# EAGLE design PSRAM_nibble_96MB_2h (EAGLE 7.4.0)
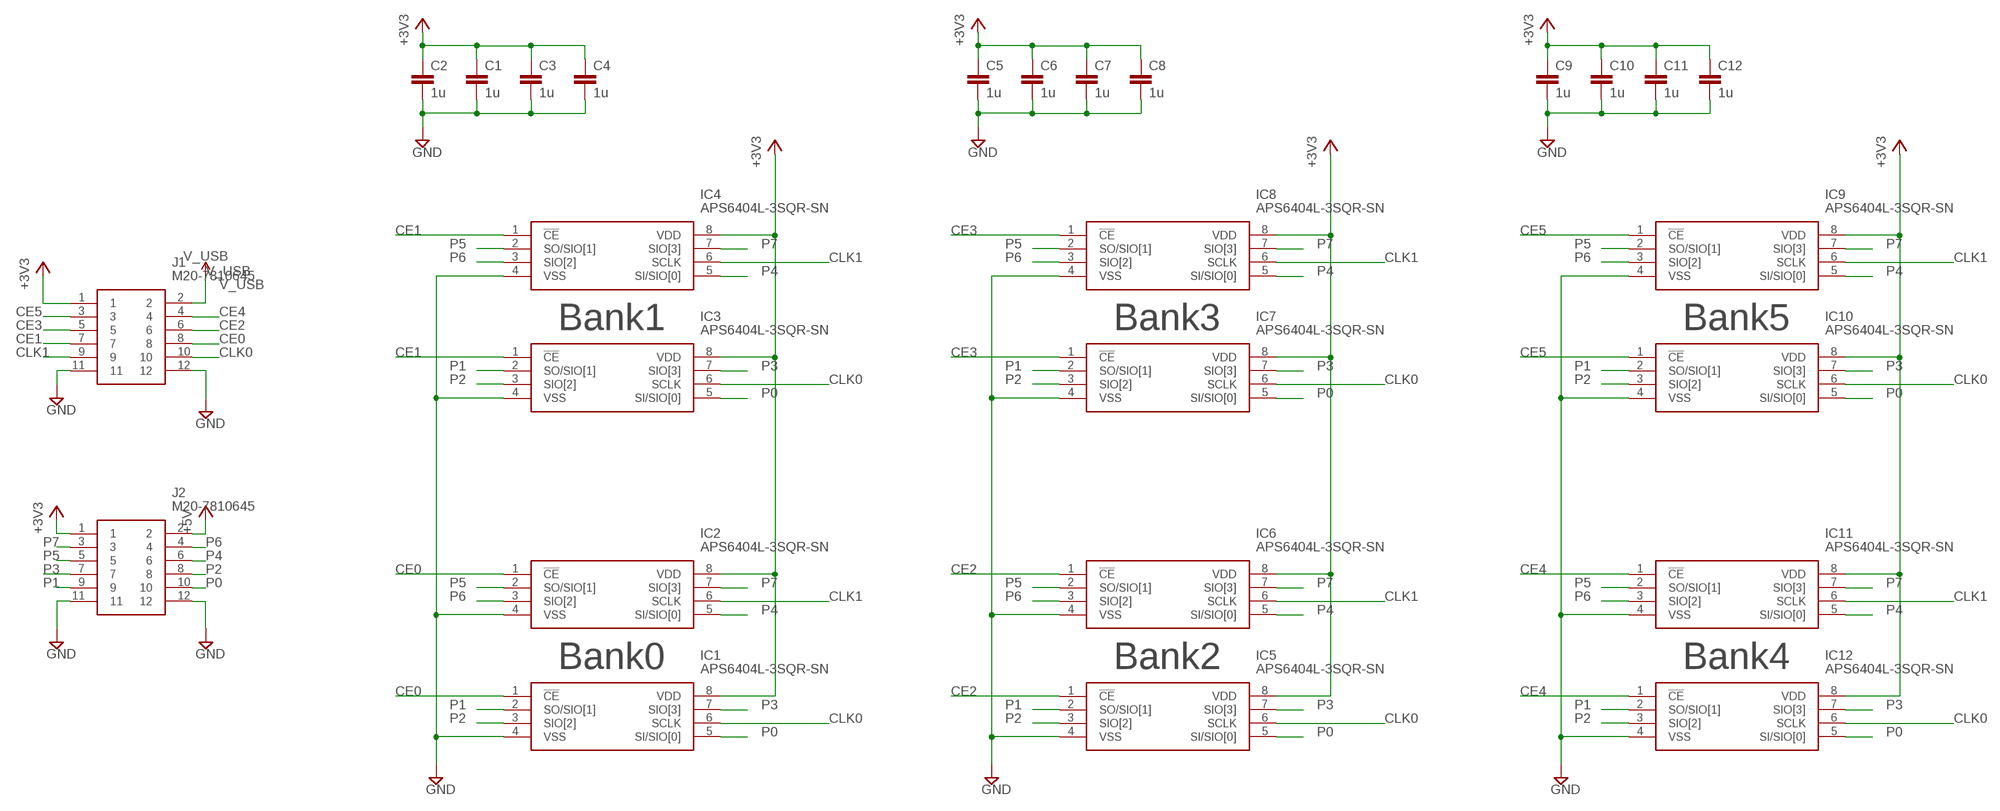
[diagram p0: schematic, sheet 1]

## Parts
C1  1u  1.0UF-25V-+80/-20(0805)  [0805@1]
C2  1u  1.0UF-25V-+80/-20(0805)  [0805@1]
C3  1u  1.0UF-25V-+80/-20(0805)  [0805@1]
C4  1u  1.0UF-25V-+80/-20(0805)  [0805@1]
C5  1u  1.0UF-25V-+80/-20(0805)  [0805@1]
C6  1u  1.0UF-25V-+80/-20(0805)  [0805@1]
C7  1u  1.0UF-25V-+80/-20(0805)  [0805@1]
C8  1u  1.0UF-25V-+80/-20(0805)  [0805@1]
C9  1u  1.0UF-25V-+80/-20(0805)  [0805@1]
C10  1u  1.0UF-25V-+80/-20(0805)  [0805@1]
C11  1u  1.0UF-25V-+80/-20(0805)  [0805@1]
C12  1u  1.0UF-25V-+80/-20(0805)  [0805@1]
IC1  APS6404L-3SQR-SN  [SOIC127P600X175-8N]
IC2  APS6404L-3SQR-SN  [SOIC127P600X175-8N]
IC3  APS6404L-3SQR-SN  [SOIC127P600X175-8N]
IC4  APS6404L-3SQR-SN  [SOIC127P600X175-8N]
IC5  APS6404L-3SQR-SN  [SOIC127P600X175-8N]
IC6  APS6404L-3SQR-SN  [SOIC127P600X175-8N]
IC7  APS6404L-3SQR-SN  [SOIC127P600X175-8N]
IC8  APS6404L-3SQR-SN  [SOIC127P600X175-8N]
IC9  APS6404L-3SQR-SN  [SOIC127P600X175-8N]
IC10  APS6404L-3SQR-SN  [SOIC127P600X175-8N]
IC11  APS6404L-3SQR-SN  [SOIC127P600X175-8N]
IC12  APS6404L-3SQR-SN  [SOIC127P600X175-8N]
J1  M20-7810645  [M207810645]
J2  M20-7810645  [M207810645]

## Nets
+3V3: C1.1 C2.1 C3.1 C4.1 C5.1 C6.1 C7.1 C8.1 C9.1 C10.1 C11.1 C12.1 IC1.8(VDD) IC2.8(VDD) IC3.8(VDD) IC4.8(VDD) IC5.8(VDD) IC6.8(VDD) IC7.8(VDD) IC8.8(VDD) IC9.8(VDD) IC10.8(VDD) IC11.8(VDD) IC12.8(VDD) J1.1 J2.1
+5V: J2.2
CE0: IC1.1(!CE) IC2.1(!CE) J1.8
CE1: IC3.1(!CE) IC4.1(!CE) J1.7
CE2: IC5.1(!CE) IC6.1(!CE) J1.6
CE3: IC7.1(!CE) IC8.1(!CE) J1.5
CE4: IC11.1(!CE) IC12.1(!CE) J1.4
CE5: IC9.1(!CE) IC10.1(!CE) J1.3
CLK0: IC1.6(SCLK) IC3.6(SCLK) IC5.6(SCLK) IC7.6(SCLK) IC10.6(SCLK) IC12.6(SCLK) J1.10
CLK1: IC2.6(SCLK) IC4.6(SCLK) IC6.6(SCLK) IC8.6(SCLK) IC9.6(SCLK) IC11.6(SCLK) J1.9
GND: C1.2 C2.2 C3.2 C4.2 C5.2 C6.2 C7.2 C8.2 C9.2 C10.2 C11.2 C12.2 IC1.4(VSS) IC2.4(VSS) IC3.4(VSS) IC4.4(VSS) IC5.4(VSS) IC6.4(VSS) IC7.4(VSS) IC8.4(VSS) IC9.4(VSS) IC10.4(VSS) IC11.4(VSS) IC12.4(VSS) J1.11 J1.12 J2.11 J2.12
P0: IC1.5(SI/SIO[0]) IC3.5(SI/SIO[0]) IC5.5(SI/SIO[0]) IC7.5(SI/SIO[0]) IC10.5(SI/SIO[0]) IC12.5(SI/SIO[0]) J2.10
P1: IC1.2(SO/SIO[1]) IC3.2(SO/SIO[1]) IC5.2(SO/SIO[1]) IC7.2(SO/SIO[1]) IC10.2(SO/SIO[1]) IC12.2(SO/SIO[1]) J2.9
P2: IC1.3(SIO[2]) IC3.3(SIO[2]) IC5.3(SIO[2]) IC7.3(SIO[2]) IC10.3(SIO[2]) IC12.3(SIO[2]) J2.8
P3: IC1.7(SIO[3]) IC3.7(SIO[3]) IC5.7(SIO[3]) IC7.7(SIO[3]) IC10.7(SIO[3]) IC12.7(SIO[3]) J2.7
P4: IC2.5(SI/SIO[0]) IC4.5(SI/SIO[0]) IC6.5(SI/SIO[0]) IC8.5(SI/SIO[0]) IC9.5(SI/SIO[0]) IC11.5(SI/SIO[0]) J2.6
P5: IC2.2(SO/SIO[1]) IC4.2(SO/SIO[1]) IC6.2(SO/SIO[1]) IC8.2(SO/SIO[1]) IC9.2(SO/SIO[1]) IC11.2(SO/SIO[1]) J2.5
P6: IC2.3(SIO[2]) IC4.3(SIO[2]) IC6.3(SIO[2]) IC8.3(SIO[2]) IC9.3(SIO[2]) IC11.3(SIO[2]) J2.4
P7: IC2.7(SIO[3]) IC4.7(SIO[3]) IC6.7(SIO[3]) IC8.7(SIO[3]) IC9.7(SIO[3]) IC11.7(SIO[3]) J2.3
V_USB: J1.2

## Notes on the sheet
- Bank1 | Bank3 | Bank5
- Bank0 | Bank2 | Bank4

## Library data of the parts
C1-C12 = SparkFun-Capacitors:1.0UF-25V-+80/-20(0805); PROD_ID: CAP-11625; VALUE: 1.0uF
IC1-IC12 = SamacSys_Parts:APS6404L-3SQR-SN: DRAM IoT RAM 64Mb QSPI (x1,x4) SDR 133/84MHz, RBX, 3V, Ind. Temp., SOP8 Source: Datasheet; DESCRIPTION: DRAM IoT RAM 64Mb QSPI (x1,x4) SDR 133/84MHz, RBX, 3V, Ind. Temp., SOP8; HEIGHT: 1.75mm; MANUFACTURER_NAME: AP Memory; MANUFACTURER_PART_NUMBER: APS6404L-3SQR-SN; MOUSER_PART_NUMBER: 878-APS6404L-3SQR-SN; MOUSER_PRICE-STOCK: https://www.mouser.co.uk/ProductDetail/AP-Memory/APS6404L-3SQR-SN?qs=IS%252B4QmGtzzqsn3S5xo%2FEEg%3D%3D
J1 J2 = SamacSys_Parts:M20-7810645: Headers & Wire Housings 6+6 DIL 2.54MM L/P SMT SKT Source: Datasheet; DESCRIPTION: Headers & Wire Housings 6+6 DIL 2.54MM L/P SMT SKT; HEIGHT: 3.7mm; MANUFACTURER_NAME: Harwin; MANUFACTURER_PART_NUMBER: M20-7810645; MOUSER_PART_NUMBER: 855-M20-7810645; MOUSER_PRICE-STOCK: https://www.mouser.co.uk/ProductDetail/Harwin/M20-7810645?qs=k41KVqW3ympKz0jQ%252Bxdz7A%3D%3D

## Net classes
1 power: width 0.254 mm
2 gnd: width 0.305 mm, drill 0.406 mm, clearance 0.203 mm

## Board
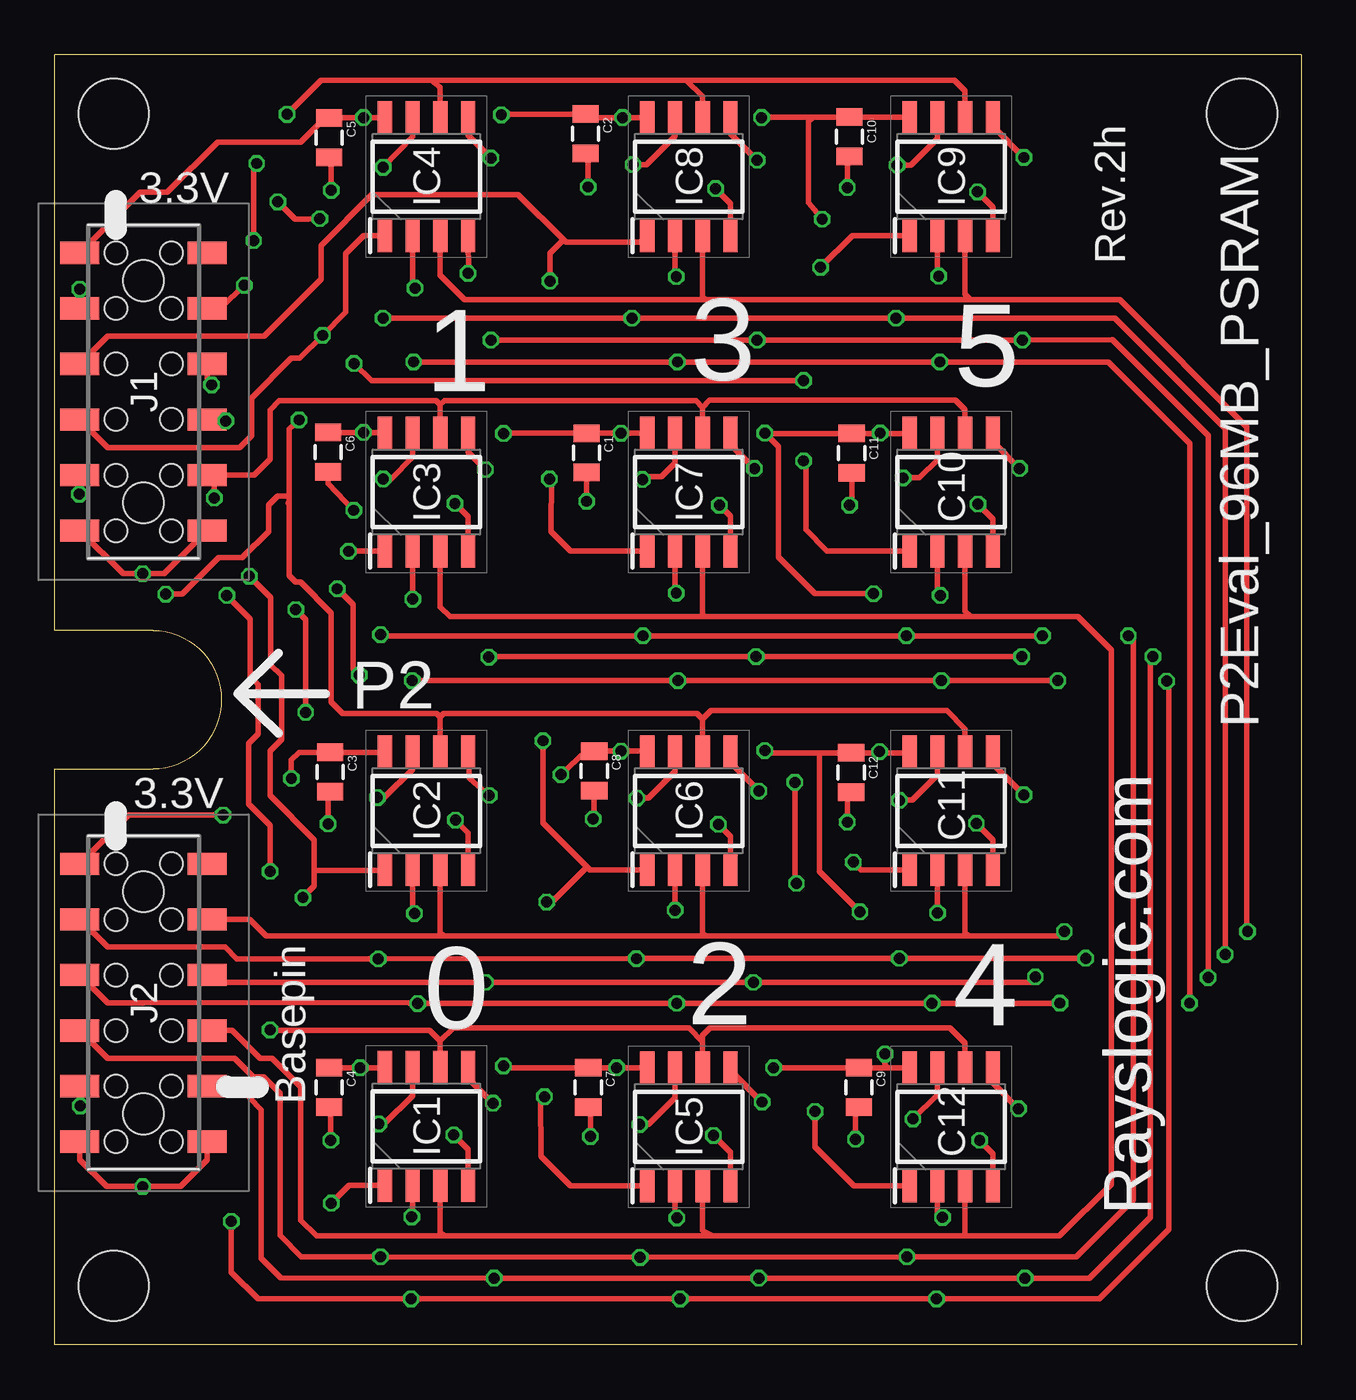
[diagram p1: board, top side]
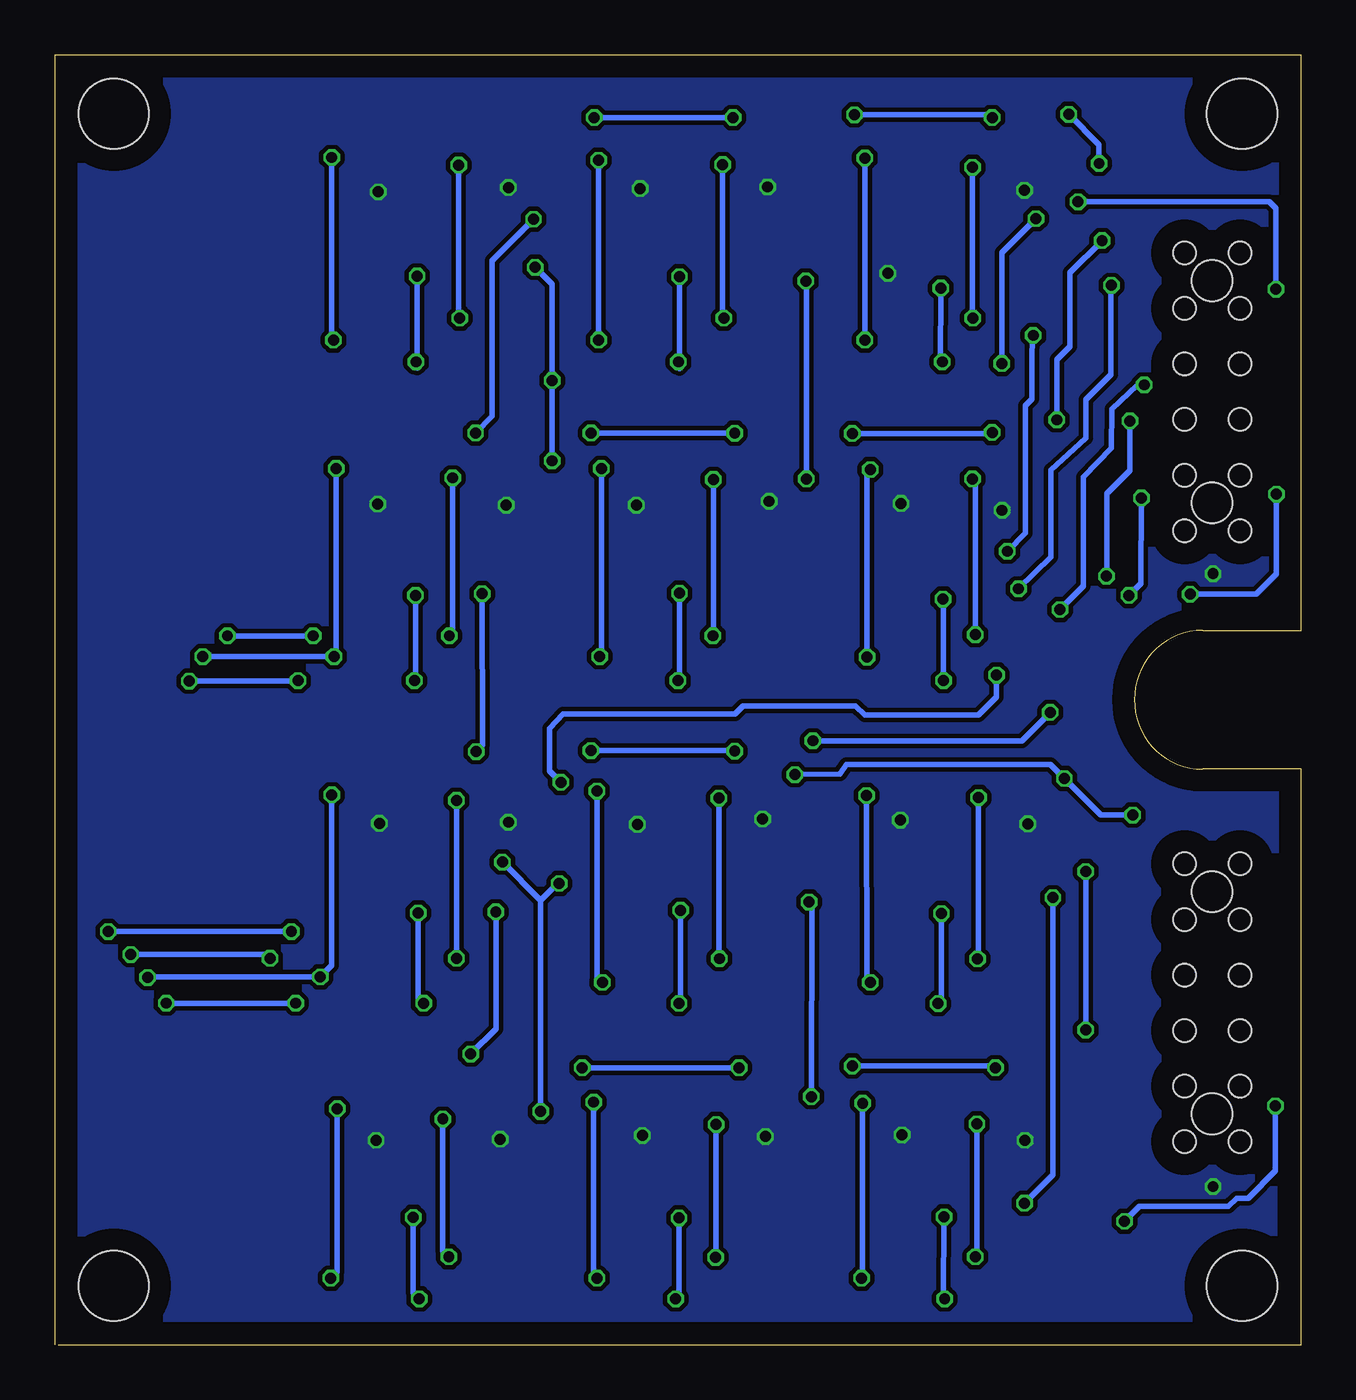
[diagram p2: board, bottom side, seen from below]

Size 57 x 59 mm. Coordinates in mm from the lower left corner, seen from the top.
Outline: 57,0 57,59 0,59 0,32.67 4.5,32.67 arc-90 7.62,29.5 arc-90 4.5,26.32 0,26.32 0,0 56.83,0
Copper layers (1*16): Top 0.035mm / dielectric 1.5mm / Bottom 0.035mm
Design rules "default *": minimum track width 10mil, minimum drill 8mil, track to track 8mil, track to pad 8mil, pad to pad 8mil, via to via 8mil, smd to smd 8mil, copper to edge 40mil, drill to drill 8mil, minimum pad ring 10mil, minimum via ring 4mil, stop-mask expansion 4mil, vias tented up to drill 0mil, thermal gap 10mil
Holes 3.2 mm at 2.7,56.3 54.3,56.3 2.7,2.7 54.3,2.7

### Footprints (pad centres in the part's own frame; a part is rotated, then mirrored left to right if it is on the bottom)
0805@1 = smd 0.8 x 1.2: 1 -0.9,0; 2 0.9,0
SOIC127P600X175-8N = smd 1.5 x 0.65: 1 -2.7,1.905; 2 -2.7,0.635; 3 -2.7,-0.635; 4 -2.7,-1.905; 5 2.7,-1.905; 6 2.7,-0.635; 7 2.7,0.635; 8 2.7,1.905
M207810645 = smd 1.02 x 1.78: 1 -6.35,-2.91; 2 -6.35,2.91; 3 -3.81,-2.91; 4 -3.81,2.91; 5 -1.27,-2.91; 6 -1.27,2.91; 7 1.27,-2.91; 8 1.27,2.91; 9 3.81,-2.91; 10 3.81,2.91; 11 6.35,-2.91; 12 6.35,2.91 | hole 1.85: -5.08,0; 5.08,0 | hole 1.02: -6.35,-1.27; -6.35,1.27; -3.81,1.27; -3.81,-1.27; -1.27,-1.27; -1.27,1.27; 1.27,1.27; 1.27,-1.27; 3.81,-1.27; 3.81,1.27; 6.35,1.27; 6.35,-1.27

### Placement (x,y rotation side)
C1  24.32,40.79 270 top
C2  24.27,55.38 270 top
C3  12.6,26.2 270 top
C4  12.55,11.78 270 top
C5  12.55,55.2 270 top
C6  12.5,40.83 270 top
C7  24.4,11.78 270 top
C8  24.68,26.25 270 top
C9  36.77,11.78 270 top
C10  36.35,55.25 270 top
C11  36.45,40.77 270 top
C12  36.42,26.18 270 top
IC1  17,10 90 top
IC2  17,24.43 90 top
IC3  17,39 90 top
IC4  17,53.42 90 top
IC5  29,9.97 90 top
IC6  29,24.43 90 top
IC7  29,39 90 top
IC8  29,53.42 90 top
IC9  41,53.42 90 top
IC10  41,39 90 top
IC11  41,24.43 90 top
IC12  41,9.97 90 top
J1  4.06,43.58 270 top
J2  4.06,15.64 270 top

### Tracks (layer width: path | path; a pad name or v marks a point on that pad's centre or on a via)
+3V3  (via drill 0.5)
  Top 0.254: IC4.8 v14.12,56.12 13.07,56.12 C5.1 12.35,56.1 11.25,55 7.45,55 5.15,52.7 3.92,52.7 J1.1 | IC8.8 v25.98,56.12 24.43,56.12 C2.1 20.43,56.28 v20.43,56.25 | IC9.8 39.07,56.15 C10.1 34.7,56.15 | IC10.8 39.07,41.67 C11.1 | IC3.8 15.07,41.73 v14.12,41.73 C6.1 | IC7.8 v25.9,41.69 C1.1 20.54,41.69 v20.52,41.67 | IC11.8 39.05,27.07 C12.1 | IC6.8 27.07,27.15 v25.9,27.15 C8.1 24.3,27.15 v23.15,26.07 | IC2.8 15.07,27.1 C3.1 11.18,27.1 10.82,26.75 v10.82,25.9 | IC1.8 15.07,12.68 v13.97,12.68 C4.1 | IC5.8 v25.7,12.68 C7.1 20.6,12.68 v20.52,12.75 | IC12.8 38.08,12.68 | 38.08,12.68 C9.1 | 34.7,56.15 32.33,56.15 v32.33,56.12 | C11.1 37.17,41.67 v37.75,41.7 | C11.1 32.5,41.67 v32.48,41.7 33.1,41.08 33.1,36.02 34.77,34.35 v37.45,34.35 | C12.1 37.52,27.07 v37.73,27.12 | v35.1,51.48 35,51.62 34.48,52.23 34.48,55.92 34.7,56.15 | C12.1 34.98,27.07 | 34.98,27.07 32.58,27.07 v32.48,27.18 | C9.1 36.83,12.72 | v36.83,19.8 34.98,21.65 34.98,27.07 | C9.1 v32.88,12.68 | v37.98,13.3 37.98,12.78 38.08,12.68 | J2.1 3.38,24.23 v7.7,24.23
  Bottom 0.254: v32.33,56.12 v25.98,56.12 | v20.43,56.25 14.12,56.25 v14.12,56.12 | v37.75,41.7 37,42.48 37,49.58 v35.1,51.48 | v32.48,41.7 v25.91,41.7 v25.9,41.69 | v20.52,41.67 14.15,41.67 v14.12,41.73 | v37.73,27.12 37.42,27.43 v37.45,34.35 | v32.48,27.18 25.93,27.18 v25.9,27.15 | v23.15,26.07 21.1,26.1 20.8,26.55 11.47,26.55 v10.82,25.9 9.15,24.23 v7.7,24.23 | v32.88,12.68 v25.7,12.68 | v20.52,12.75 14.05,12.75 v13.97,12.68 | v36.83,19.8 36.83,14.45 v37.98,13.3
CE0  (via drill 0.5)
  Top 0.254: 11.88,21.7 15.07,21.7 IC2.1 | IC1.1 13.47,7.3 v12.65,6.47 | v11.35,20.45 11.88,20.98 11.88,21.7 | J1.8 6.99,42.33 v7.83,42.25 | 11.88,21.7 11.88,23.1 9.85,25.12 9.85,27.15 10.38,27.68 10.38,30.6 9.88,31.1 9.88,34.17 v8.9,35.15
  Bottom 0.254: v12.65,6.47 11.35,7.78 v11.35,20.45 | v8.9,35.15 8.88,35.08 8.88,38.92 7.83,39.98 v7.83,42.25
CE1  (via drill 0.5)
  Top 0.254: IC4.1 14.12,50.73 13.3,49.9 13.3,47.23 v12.25,46.16 11.21,45.12 10.82,45.12 9,43.3 9,41.58 8.46,41.04 2.43,41.04 J1.7 | IC3.1 13.35,36.3 v13.44,36.29
  Bottom 0.254: v12.25,46.16 12.31,45.44 12.31,43.24 12.6,42.95 12.6,37.12 v13.44,36.29
CE2  (via drill 0.5)
  Top 0.254: v22.32,27.62 22.32,23.88 24.35,21.85 | 24.35,21.85 24.48,21.73 IC6.1 | IC5.1 23.6,7.28 22.25,8.62 22.23,11.35 v22.4,11.35 | v22.5,20.25 22.75,20.25 24.35,21.85 | J1.6 6.97,44.1 v7.17,43.9 | v11.03,33.62 11.47,33.17 v11.47,28.93
  Bottom 0.254: v22.4,11.35 22.38,20.12 v22.5,20.25 | v7.17,43.9 7.5,43.9 8.65,42.8 8.68,41 9.95,39.67 9.95,34.7 v11.03,33.62 | v11.47,28.93 12.78,27.62 v22.32,27.62
CE3  (via drill 0.5)
  Top 0.254: 23.26,50.54 21.2,52.6 14.5,52.6 12.18,50.27 12.18,48.73 9.57,46.12 2.42,46.12 J1.5 | 23.26,50.54 23.38,50.42 26.8,50.42 IC8.1 | IC7.1 23.6,36.3 22.7,37.2 22.73,39.77 v22.62,39.6 | v22.65,48.65 22.65,49.92 23.26,50.54
  Bottom 0.254: v22.62,39.6 22.62,48.62 v22.65,48.65
CE4  (via drill 0.5)
  Top 0.254: IC11.1 36.88,21.73 v36.52,22.07 | v34.77,10.68 34.77,9.05 36.55,7.28 IC12.1 | v33.92,21.1 33.85,21.18 v33.85,25.73 | v8.68,48.45 7.62,47.42 J1.4 | v12.93,34.58 13.65,33.85 13.65,30.9 v13.93,30.62
  Bottom 0.254: v36.52,22.07 34.77,20.32 | 34.77,20.32 v34.77,10.68 | 34.77,20.32 34,21.1 v33.92,21.1 | v33.85,25.73 34.38,26.25 34.38,28.18 33.75,28.85 25.9,28.85 25.52,29.23 20.38,29.23 19.95,28.8 14.75,28.8 13.93,29.62 v13.93,30.62 | v8.68,48.45 8.7,48.3 8.7,44.38 9.85,43.23 9.85,41.48 11.45,40 11.45,36.02 v12.93,34.58
CE5  (via drill 0.5)
  Top 0.254: IC10.1 35.33,36.3 34.35,37.27 34.35,40.33 v34.25,40.42 | v35.02,49.27 36.48,50.73 IC9.1 | v12.12,51.5 11.6,51.49 10.99,51.49 v10.2,52.27 | v13.69,44.88 14.49,44.1 v34.25,44.1 | v1.15,48.27 J1.3
  Bottom 0.254: v35.02,49.27 34.25,48.5 v34.25,44.1 v34.25,40.42 | v12.12,51.5 13.69,49.95 v13.69,44.88 | v10.2,52.27 1.45,52.27 1.15,51.98 v1.15,48.27
CLK0  (via drill 0.5)
  Top 0.254: 17.64,42.99 17.45,43.17 10.28,43.17 9.85,42.75 9.85,40.5 9.12,39.77 J1.10 | 17.64,42.99 IC3.6 | IC7.6 29.64,42.87 | 29.64,42.87 29.32,43.17 17.82,43.17 17.64,42.99 | IC10.6 41.63,42.77 41.2,43.2 29.95,43.2 29.64,42.87 | IC1.6 17.64,13.89 | 17.64,13.89 17.15,14.38 9.88,14.38 v9.85,14.4 | IC12.6 41.63,13.81 40.95,14.5 29.98,14.5 29.64,14.16 IC5.6 29.64,13.87 29,14.5 18.25,14.5 17.64,13.89 | 6.9,39.77 J1.10 | J1.10 7.3,39.45 v7.3,38.73 | v9.85,21.65 9.85,23.75 8.88,24.73 8.88,27.5 9.3,27.93 9.3,30.2 8.95,30.55 8.95,33.2 8.03,34.1 v7.88,34.27
  Bottom 0.254: v9.85,14.4 v9.85,21.65 | v7.3,38.73 7.33,34.83 v7.88,34.27
CLK1  (via drill 0.5)
  Top 0.254: 10.72,38.83 10.72,41.88 v11.18,42.3 | 10.72,38.83 10.72,38.54 | 10.72,38.54 10.72,35.17 11.03,34.88 11.25,34.88 12.65,33.48 12.65,29.4 13.18,28.88 17.48,28.88 17.64,28.71 | 17.64,28.71 IC2.6 | IC6.6 29.64,28.61 | 29.64,28.61 29.38,28.88 17.8,28.88 17.64,28.71 | IC11.6 41.63,28.16 40.8,29 30.02,29 29.64,28.61 | v10.62,56.27 12.18,57.83 17.23,57.83 | 17.23,57.83 17.64,57.52 IC4.6 | IC8.6 29.64,57.09 28.86,57.84 | 28.86,57.84 28.85,57.83 17.23,57.83 | IC9.6 41.63,57.34 41.15,57.83 29.1,57.83 28.86,57.84 | v9.1,50.5 9.1,53.89 v9.24,54.02 | 10.69,38.5 10.72,38.54 | J1.9 1.12,39.74 v1.12,38.9 | 10.72,38.83 10.2,38.83 9.78,38.4 9.78,37.2 8.57,36 7.5,36 5.83,34.33 v5.08,34.33
  Bottom 0.254: 10.7,56.17 v10.62,56.27 9.24,54.89 v9.24,54.02 | v1.12,38.9 1.12,35.25 2.05,34.33 v5.08,34.33 5.12,34.35 | v11.18,42.3 11.18,45.05 10.57,45.65 10.57,49.02 v9.1,50.5
GND  (via drill 0.5)
  Top 0.254: C5.2 12.65,54.2 v12.65,52.8 | v18.9,49 18.93,48.95 IC4.4 | C2.2 24.4,54.36 v24.4,52.95 | v30.23,52.88 30.91,52.2 IC8.4 | C10.2 36.25,54.25 v36.25,52.92 | v42.2,52.73 42.91,52.02 IC9.4 | v18.3,38.48 18.91,37.87 IC3.4 | v13.68,38.16 12.5,39.38 C6.2 | C1.2 v24.32,38.58 | IC7.4 30.91,37.9 v30.4,38.4 | C11.2 36.45,38.5 v36.35,38.4 | v42.23,38.45 42.91,37.77 IC10.4 | C3.2 12.5,25.2 v12.5,23.82 | v18.32,24 18.91,23.42 IC2.4 | v24.62,24.05 24.68,24.1 C8.2 | v30.35,23.8 30.91,23.25 IC6.4 | C12.2 36.25,25.1 v36.25,23.9 | v42.15,23.85 42.91,23.09 IC11.4 | C4.2 12.62,10.8 v12.62,9.35 | v18.25,9.6 18.91,8.95 IC1.4 | C7.2 24.5,10.78 v24.5,9.53 | v30.12,9.57 30.91,8.79 IC5.4 | C9.2 36.62,10.72 v36.62,9.4 | v42.3,9.35 42.91,8.74 IC12.4 | J1.11 3.13,35.26 v4.03,35.26 5,35.26 J1.12 | J2.11 1.15,8.47 2.39,7.24 v4.03,7.24 5.76,7.24 6.97,8.45 J2.12
  pour Bottom: 1.06,55.48 4.15,58.25 53.43,58.17 55.91,55.1 55.81,4.52 53.7,1.25 3.15,1.25 1.27,4.49
P0  (via drill 0.5)
  Top 0.254: IC1.5 18.91,12.2 v20.05,11.05 | IC5.5 30.91,12.54 v32.35,11.1 | IC12.5 42.91,11.97 v44.08,10.8 | v50.23,31.48 50.1,31.35 50.1,5.83 47.33,3.05 v44.38,3.05 v32.2,3.05 v20.1,3.05 10.32,3.08 9.45,3.95 9.45,10.75 8.39,11.83 J2.10 | v44.23,31.48 v32.08,31.48 19.88,31.48 v19.85,31.45 | v19.7,40.02 18.91,40.82 IC3.5 | IC7.5 30.91,41.17 v32,40.08 | IC10.5 42.91,41.3 v44.12,40.08
  Bottom 0.254: v20.05,11.05 20.05,3.1 v20.1,3.05 | v32.35,11.1 32.35,3.2 v32.2,3.05 | v44.08,10.8 44.08,3.35 v44.38,3.05 | v50.23,31.48 v44.23,31.48 44.12,31.57 v44.12,40.08 | v19.85,31.45 19.85,39.88 v19.7,40.02 | v32,40.08 32,31.55 v32.08,31.48
P1  (via drill 0.5)
  Top 0.254: IC1.2 16.36,5.82 v16.32,5.85 | IC5.2 28.36,5.88 v28.45,5.8 | IC12.2 40.37,6.01 v40.6,5.83 | v50.85,30.35 50.95,30.27 50.95,5.28 47.77,2.1 v40.33,2.1 v28.6,2.1 v16.3,2.1 9.3,2.1 8.07,3.33 v8.07,5.65 | v45.88,30.38 v40.55,30.38 v28.5,30.38 v16.35,30.38 | v16.38,34.1 16.38,36.29 IC3.2 | IC7.2 28.36,34.44 v28.43,34.38 | IC10.2 40.37,34.41 v40.5,34.27 | J2.9 1.15,10.95 v1.18,10.93
  Bottom 0.254: v16.32,5.85 16.35,2.15 v16.3,2.1 | v28.45,5.8 28.45,2.25 v28.6,2.1 | v40.6,5.83 40.6,2.38 v40.33,2.1 | v50.85,30.35 45.9,30.35 v45.88,30.38 | v16.35,30.38 16.35,34.08 v16.38,34.1 | v28.43,34.38 28.43,30.45 v28.5,30.38 | v40.5,34.27 40.5,30.43 v40.55,30.38 | v1.18,10.93 1.18,7.95 2.42,6.7 2.95,6.7 3.33,6.33 7.4,6.33 v8.07,5.65
P2
  Top 0.254: 17.82,4.97 11.97,4.97 11.25,5.7 11.25,11.8 9.95,13.1 9.4,13.1 8.13,14.37 J2.8 | 17.82,4.97 30.12,4.97 | 30.12,4.97 41.7,4.97 | 41.7,4.97 45.95,4.97 48.33,7.35 48.33,31.77 46.8,33.3 41.9,33.3 | IC1.3 17.64,5.17 17.82,4.97 | IC5.3 29.64,5.24 30.12,4.97 | IC12.3 41.63,5.04 41.7,4.97 | 41.9,33.3 29.73,33.3 | 29.73,33.3 18.07,33.3 17.64,33.74 IC3.3 | IC7.3 29.64,33.39 29.73,33.3 | IC10.3 41.63,33.56 41.9,33.3
P3  (via drill 0.5)
  Top 0.254: IC1.7 16.36,11.39 15.07,10.1 v14.82,10.1 | IC5.7 28.36,11.29 27.15,10.07 v26.75,10.07 | IC12.7 40.37,11.44 v39.25,10.32 | v49.1,32.42 49.33,32.2 49.33,6.62 46.73,4.03 v38.98,4.03 v26.77,4 v14.9,4.03 11.28,4.03 10.3,5 10.3,11.5 9.55,12.25 9.07,12.25 8.22,13.1 2.43,13.1 J2.7 | v45.17,32.42 v38.95,32.42 v26.9,32.42 14.95,32.42 v14.9,32.48 | v15.03,39.6 15.38,39.6 16.36,40.59 IC3.7 | IC7.7 28.36,40.31 27.75,39.7 27,39.7 v26.88,39.58 | IC10.7 40.37,40.47 39.55,39.65 v38.8,39.65
  Bottom 0.254: v14.82,10.1 14.82,4.22 v14.9,4.03 | v26.75,10.07 26.75,4.03 v26.77,4 | v39.25,10.32 39.25,4.3 v38.98,4.03 | v49.1,32.42 v45.17,32.42 | v14.9,32.48 14.9,39.48 v15.03,39.6 | v26.88,39.58 26.88,32.48 v26.9,32.42 | v38.8,39.65 38.8,32.73 v38.95,32.42
P4  (via drill 0.5)
  Top 0.254: v44.85,16.82 44.62,16.57 v31.95,16.57 v19.7,16.57 7.78,16.57 7.44,16.91 J2.6 | IC2.5 18.98,25.89 v19.88,25.12 | IC4.5 18.91,55.32 v19.95,54.27 | v19.95,45.95 v32.12,45.95 v44.25,45.95 48.38,45.98 52.75,41.58 v52.75,16.8 | IC6.5 30.91,26.62 v32.2,25.32 | IC11.5 42.91,26.57 v44.33,25.15 | IC8.5 30.91,55.4 v32.12,54.17 | IC9.5 42.91,55.72 v44.33,54.3
  Bottom 0.254: v52.75,16.8 52.73,16.82 v44.85,16.82 44.33,17.35 v44.33,25.15 | v19.88,25.12 19.85,16.73 v19.7,16.57 | v19.95,54.27 v19.95,45.95 | v32.2,25.32 32.2,16.82 v31.95,16.57 | v32.12,54.17 v32.12,45.95 | v44.33,54.3 44.33,45.92 v44.25,45.95
P5  (via drill 0.5)
  Top 0.254: v16.6,15.61 v28.45,15.61 | v28.45,15.61 39.8,15.62 | 39.8,15.62 v40.12,15.62 | v40.12,15.62 v45.98,15.62 | IC2.2 16.36,19.81 v16.45,19.73 | v16.6,15.61 16.23,15.61 | IC4.2 16.36,48.47 v16.48,48.33 | v16.41,44.95 v28.48,44.95 v40.48,44.95 48.17,44.95 51.9,41.23 v51.9,15.62 | IC6.2 28.36,19.89 v28.38,19.88 | v28.45,15.61 27.98,15.61 | IC11.2 40.37,19.76 v40.38,19.75 | v40.12,15.62 39.8,15.62 | 39.8,15.62 | IC8.2 28.36,48.91 v28.43,48.85 | IC9.2 40.37,48.94 v40.42,48.88 | v16.6,15.61 16.55,15.65 4.06,15.64 2.43,15.64 J2.5
  Bottom 0.254: v45.98,15.62 v51.9,15.62 | v16.45,19.73 16.45,15.76 v16.6,15.61 | v16.48,48.33 16.49,44.89 v16.41,44.95 | v28.38,19.88 28.38,15.69 v28.45,15.61 | v40.38,19.75 40.38,15.87 v40.12,15.62 | v28.43,48.85 28.43,44.65 v28.48,44.95 | v40.42,48.88 40.42,44.67 v40.48,44.95
P6  (via drill 0.5)
  Top 0.254: 17.8,18.7 9.68,18.7 8.92,19.45 J2.4 | 17.8,18.7 29.77,18.7 | 29.77,18.7 41.8,18.7 | 41.8,18.7 45.98,18.7 v46.17,18.9 | IC2.3 17.64,18.86 17.8,18.7 | IC4.3 17.64,48.91 18.75,47.8 29.77,47.8 | 29.77,47.8 41.88,47.8 | v54.55,18.9 54.52,18.93 54.52,41.98 48.7,47.8 41.88,47.8 | IC6.3 29.64,18.84 29.77,18.7 | IC11.3 41.63,18.86 41.8,18.7 | IC8.3 29.64,47.94 29.77,47.8 | IC9.3 41.63,48.04 41.88,47.8
  Bottom 0.254: v46.17,18.9 v54.55,18.9
P7  (via drill 0.5)
  Top 0.254: v26.6,17.66 v14.8,17.65 8.32,17.65 7.8,18.19 2.42,18.19 J2.3 | v26.6,17.66 26.75,17.66 | 26.75,17.66 v38.62,17.67 | v38.62,17.67 v47.15,17.68 | IC2.7 16.36,26.32 15.07,25.02 v14.75,25.02 | IC4.7 16.36,55.24 v15.03,53.85 | v15.01,46.95 v26.4,46.95 v38.48,46.95 48.48,46.95 53.52,41.9 v53.52,17.85 | IC6.7 28.36,26.21 27.15,25 v26.62,25 | v26.6,17.66 26.75,17.66 | 26.75,17.66 | IC11.7 40.37,26.07 39.23,24.93 38.65,24.93 v38.62,24.9 | v38.62,17.67 38.4,17.67 | IC8.7 28.36,55.27 27.07,53.98 v26.45,53.98 | IC9.7 40.37,55.16 39.15,53.95 v38.52,53.95
  Bottom 0.254: v47.15,17.68 47.33,17.85 v53.52,17.85 | v14.75,25.02 14.75,17.8 v14.8,17.65 | v15.03,53.85 15.03,47.05 v15.01,46.95 | v26.62,25 26.62,17.68 v26.6,17.66 | v38.62,24.9 v38.62,17.67 | v38.62,17.67 | v26.45,53.98 26.45,47 v26.4,46.95 | v38.52,53.95 38.52,47 v38.48,46.95

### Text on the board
tPlace: 3.3V | Rev.2h | 1 | 3 | 5 | P2 | P2Eval_96MB_PSRAM | 3.3V | 2 | 4 | 0 | Basepin | Rayslogic.com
